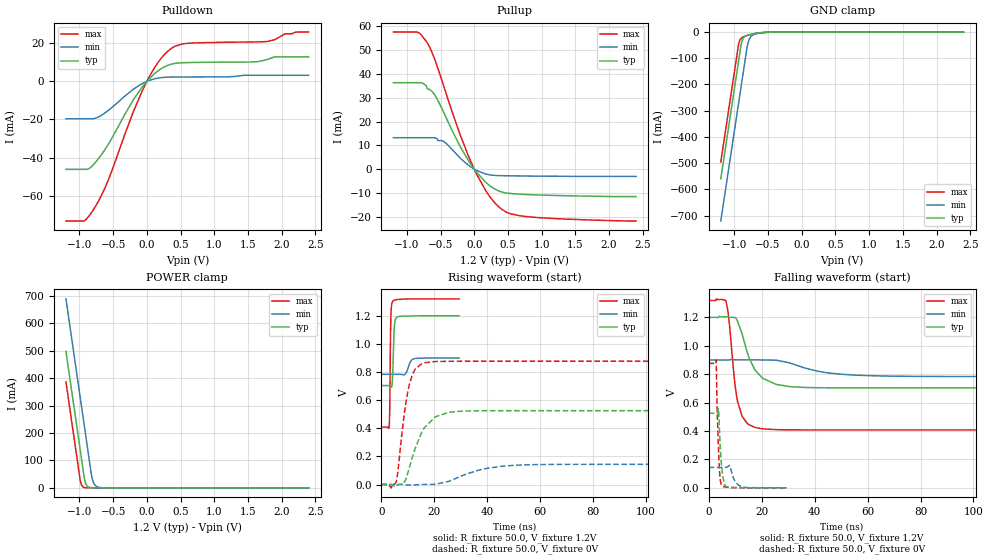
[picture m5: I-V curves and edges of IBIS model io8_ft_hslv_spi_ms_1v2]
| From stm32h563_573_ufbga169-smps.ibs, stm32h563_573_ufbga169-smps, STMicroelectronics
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[Model]   io8_ft_hslv_spi_ms_1v2
Model_type I/O
Polarity   Non-Inverting
Enable   Active-Low
| CAP_THRESHOLD on pad IOFT is "UDTCAPC" :
| Rising=20.0% of vddiom   Falling=80.0% of vddiom
| C_comp min and max val. don't necessarily correlate with the min and max pvt
| but are the smallest and greatest pad capacitance found.
| var   typ   min   max
C_comp   4.03050pF  3.93195pF  4.03600pF
|C_comp_pullup   2.46600pF  2.28050pF  2.18970pF
|C_comp_pulldown   1.56450pF  1.65145pF  1.84630pF
Vinl = 270.0mV
Vinh = 924.0mV
Vmeas = 600.0mV   | Reference voltage for timing measurements
Cref  = 50.0pF   | Timing specification test load capacitance value
Rref  = 100.0MOhm   | Timing specification test load resistance value
Vref  = 600.0mV   | Timing specification test load voltage
[Model Spec]
| TIME_THRESHOLD on pin ZIV11 is "CMOS" :
| Rising=40.0% of vdd   Falling=60.0% of vdd
Vinl 447.80000mV 344.80000mV 489.80000mV
Vinh 733.20000mV 535.20000mV 813.20000mV
| variable   typ   min   max
[Temperature Range] 25.0 125.0 -40.0
| variable   typ   min   max
[Voltage Range] 1.2V 900.0mV 1.32V
| variable   typ   min   max
[POWER Clamp Reference] 1.2V 900.0mV 1.32V
| variable   typ   min   max
[GND Clamp Reference] 0V 0V 0V
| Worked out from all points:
|   slope of the pulldown table from 0 to 0.18 V, typ, clamps not added: 30.6 ohm
|   slope of the pullup table from 0 to 0.18 V, typ, clamps not added: 31.3 ohm
|   GND clamp passes 1 mA (typ) near -0.52 V on its own axis
|   POWER clamp passes 1 mA (typ) near -0.84 V on its own axis
|   rising waveform, R_fixture 50.0, V_fixture 1.2V: 20-80 % time 523ps typ, 1.44ns min, 331ps max; typ from 0.704 V to 1.2 V
|   falling waveform, R_fixture 50.0, V_fixture 1.2V: 20-80 % time 6.5ns typ, 15.2ns min, 3.28ns max; typ from 1.2 V to 0.704 V
|   rising waveform, R_fixture 50.0, V_fixture 0V: 20-80 % time 6.75ns typ, 13.6ns min, 3.74ns max; typ from 0 V to 0.525 V
|   falling waveform, R_fixture 50.0, V_fixture 0V: 20-80 % time 1.15ns typ, 2.1ns min, 895ps max; typ from 0.525 V to 0 V
[POWER Clamp]
-1.2V     497.8mA    689.2mA    386.5mA
-990mV    140.8mA    332.2mA    29.53mA
-980mV    123.8mA    315.2mA    17.95mA
-960mV    89.81mA    281.2mA    6.634mA
-930mV    38.81mA    230.2mA    1.49mA
-900mV    12.07mA    179.2mA    334.8uA
-870mV    3.756mA    128.2mA    75.22uA
-820mV    536.4uA    44.98mA    6.246uA
-790mV    166.9uA    18.76mA    1.403uA
-750mV    35.18uA    5.846mA    191.9nA
-590mV    70.47nA    54.99uA    202.5pA
2.4V      0A         0A         0A
[GND Clamp]
-1.2V     -559.6mA   -720.6mA   -495.5mA
-940mV    -117.6mA   -278.6mA   -53.46mA
-930mV    -100.6mA   -261.6mA   -41.27mA
-900mV    -50.49mA   -210.6mA   -24.86mA
-880mV    -31.4mA    -176.6mA   -20.57mA
-850mV    -18.9mA    -125.6mA   -16.88mA
-810mV    -12.57mA   -58.3mA    -13.49mA
-780mV    -10.11mA   -29.57mA   -11.38mA
-740mV    -7.754mA   -14.31mA   -8.91mA
-640mV    -3.713mA   -4.821mA   -4.078mA
-390mV    -82.2uA    -288.6uA   -29.73uA
2.4V      3.859nA    727.5nA    172.3pA
| variable   typ   min   max
[Pullup Reference] 1.2V 900.0mV 1.32V
| variable   typ   min   max
[Pulldown Reference] 0V 0V 0V
[Pullup]
-1.2V     36.36mA    13.24mA    57.67mA
-840mV    36.36mA    13.24mA    57.6mA
-750mV    35.91mA    13.24mA    55.07mA
-700mV    33.93mA    13.24mA    53.25mA
-600mV    31.73mA    13.24mA    47.16mA
-450mV    23.69mA    11.59mA    34.67mA
-200mV    9.064mA    4.397mA    13.74mA
0V        7.46pA     726pA      4.231pA
200mV     -6.245mA   -2.229mA   -10.29mA
400mV     -9.506mA   -2.731mA   -16.68mA
790mV     -10.67mA   -2.88mA    -19.97mA
2.4V      -11.52mA   -3.045mA   -21.79mA
[Pulldown]
-1.2V     -46.17mA   -19.62mA   -73.27mA
-930mV    -46.17mA   -19.62mA   -73.17mA
-770mV    -42.8mA    -19.41mA   -66.04mA
-570mV    -32.88mA   -15.18mA   -51.58mA
-200mV    -9.658mA   -4.083mA   -15.89mA
-80mV     -3.488mA   -1.363mA   -5.887mA
140mV     4.817mA    1.546mA    8.585mA
340mV     8.782mA    2.251mA    16.66mA
540mV     9.805mA    2.305mA    19.74mA
1.79V     11.49mA    3.197mA    20.93mA
2.05V     12.83mA    3.197mA    24.95mA
2.4V      12.83mA    3.197mA    25.89mA
[Ramp]
dV/dt_r 315.16876mV/6.48706ns 86.12196mV/13.51283ns 525.78562mV/3.72534ns
dV/dt_f 297.79741mV/6.20629ns 69.92036mV/15.14557ns 547.13927mV/3.20437ns
R_load = 50.0
| Removed startup time: 0s 0s 0s  .
| Removed end time: 29.4ns.
[Rising Waveform]
R_fixture   = 50.0
V_fixture   = 1.2V
V_fixture_min = 900.0mV
V_fixture_max = 1.32V
0s        703.7mV    783.5mV    408.1mV
3ns       703.9mV    783.4mV    411.1mV
3.2ns     704.1mV    783.5mV    530.9mV
3.45ns    702.6mV    783.5mV    980.1mV
3.6ns     699.3mV    783.5mV    1.161V
4.3ns     772.6mV    783.5mV    1.302V
5ns       1.134V     783.5mV    1.31V
6ns       1.191V     783.5mV    1.315V
12.6ns    1.199V     894.9mV    1.32V
29.4ns    1.2V       899.6mV    1.32V
| Removed startup time: 0s 0s 0s  .
| Removed end time: 249.4ns.
[Falling Waveform]
R_fixture   = 50.0
V_fixture   = 1.2V
V_fixture_min = 900.0mV
V_fixture_max = 1.32V
0s        1.2V       900mV      1.32V
6.5ns     1.205V     899.9mV    1.317V
7.55ns    1.203V     899.7mV    1.202V
9.7ns     1.199V     901.7mV    770.1mV
10.95ns   1.172V     900.9mV    605.5mV
12.65ns   1.083V     900.9mV    503.6mV
17.5ns    829.2mV    901mV      425.5mV
25.45ns   728.3mV    899.1mV    409.7mV
36.4ns    706.7mV    843.1mV    408.2mV
249.4ns   703.7mV    783.5mV    408.1mV
| Removed startup time: 0s 0s 0s  .
| Removed end time: 249.4ns.
[Rising Waveform]
R_fixture   = 50.0
V_fixture   = 0V
V_fixture_min = 0V
V_fixture_max = 0V
0s        166.4nV    850.9nV    114.4nV
5.6ns     -9.091mV   -3.26uV    16.63mV
8.6ns     12.29mV    -509uV     486.4mV
10.6ns    118.6mV    -3.436mV   709.8mV
12.8ns    256.4mV    -2.69mV    820mV
16.3ns    404.5mV    352.8uV    865.2mV
25.5ns    512.8mV    22.36mV    875.9mV
37.8ns    524.4mV    106.7mV    876.2mV
56ns      525.1mV    140.5mV    876.3mV
249.4ns   525.3mV    143.5mV    876.3mV
| Removed startup time: 0s 0s 0s  .
| Removed end time: 29.4ns.
[Falling Waveform]
R_fixture   = 50.0
V_fixture   = 0V
V_fixture_min = 0V
V_fixture_max = 0V
0s        525.3mV    143.6mV    876.3mV
2.8ns     525.4mV    143.6mV    901mV
3.25ns    527.3mV    143.6mV    522.1mV
3.65ns    558.4mV    143.6mV    306.3mV
3.9ns     489mV      143.6mV    195.4mV
4.35ns    299.4mV    143.6mV    62.62mV
4.95ns    143.2mV    143.6mV    18.56mV
6.6ns     9.649mV    143.9mV    4.761mV
12.6ns    1.357mV    7.745mV    401.8uV
29.4ns    28.13uV    458.1uV    1.646uV
